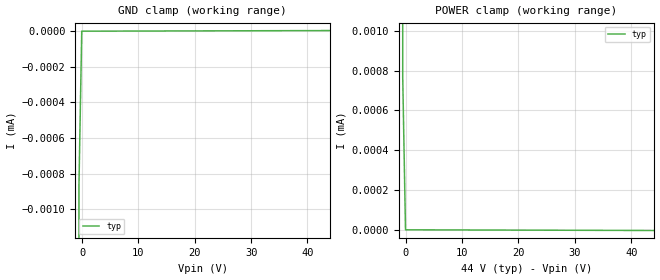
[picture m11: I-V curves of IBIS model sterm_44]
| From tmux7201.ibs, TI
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| sterm_44
[Model]   sterm_44
Model_type   Terminator
|   typ   min   max
C_comp   4.014581e-11   NA   NA
[Voltage Range]   44   NA   NA
[Temperature Range]   27   NA   NA
[Power Clamp Reference]   44   NA   NA
[GND Clamp Reference]   0   NA   NA
[GND Clamp]
|   Voltage   I(typ)   I(min)   I(max)
-5V       -10.55A    NA         NA
-1.04V    -180.8mA   NA         NA
-545.5mV  -860.9nA   NA         NA
-50.51mV  -1.726nA   NA         NA
44V       1.721nA    NA         NA
[POWER Clamp]
|   Voltage   I(typ)   I(min)   I(max)
-5V       13.28A     NA         NA
-1.04V    178.1mA    NA         NA
-545.5mV  769.7nA    NA         NA
-50.5mV   1.725nA    NA         NA
44V       -1.722nA   NA         NA
